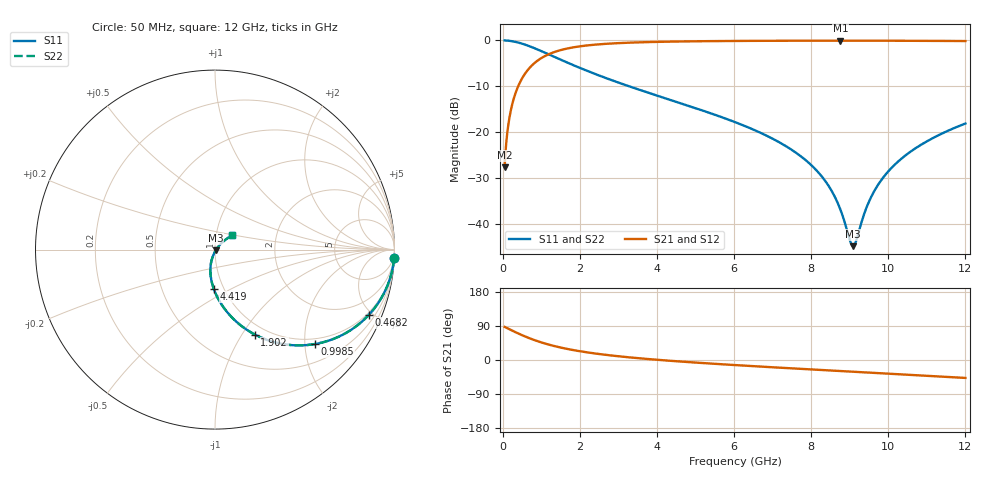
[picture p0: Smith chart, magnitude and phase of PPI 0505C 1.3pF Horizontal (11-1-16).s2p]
# MHz S MA R 50
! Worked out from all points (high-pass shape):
!   1601 points, 50 MHz to 12 GHz, reference 50 ohm
!   highest |S21| = -0.05 dB at 8.759 GHz (marker M1); lowest = -27.6 dB at 50 MHz (marker M2)
!   |S21| within 3 dB of the highest: 1.182 GHz to end of sweep
!   lowest |S11| = -44.8 dB at 9.087 GHz (marker M3), VSWR 1.01, Z = 50.5 - j0.307 ohm
!   |S11| at or under -10 dB: 3.281 GHz to end of sweep
!   |S22| runs from -44.8 to 0.0 dB; largest |S21 - S12| = 0
!   S11 on the Smith chart (normalised r, x): 50 MHz: 1, -45; 468.2 MHz: 0.87, -4.78; 998.5 MHz: 0.87, -2.23; 1.902 GHz: 0.88, -1.14; 4.419 GHz: 0.90, -0.41; 12 GHz: 1.20, +0.19
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50  0.9991 -2.6  0.0415 87.4  0.0415 87.4  0.9991 -2.6
147.0938  0.9926 -7.5  0.1213 82.5  0.1213 82.5  0.9926 -7.5
214.3125  0.9844 -10.8  0.1753 79.1  0.1753 79.1  0.9844 -10.8
468.25  0.9315 -22.9  0.363 67.0  0.363 67.0  0.9315 -22.9
998.5312  0.7665 -43.3  0.6407 46.6  0.6407 46.6  0.7665 -43.3
1902.25  0.5227 -64.9  0.85 24.9  0.85 24.9  0.5227 -64.9
2044.156  0.4938 -67.3  0.867 22.5  0.867 22.5  0.4938 -67.3
2888.125  0.3613 -78.4  0.9293 11.1  0.9293 11.1  0.3613 -78.4
4038.312  0.2479 -88.9  0.965 0.3  0.965 0.3  0.2479 -88.9
4419.219  0.2199 -91.7  0.9715 -2.6  0.9715 -2.6  0.2199 -91.7
6025  0.1289 -101.5  0.9869 -13.4  0.9869 -13.4  0.1289 -101.5
7205.062  0.07639 -106.7  0.9918 -20.4  0.9918 -20.4  0.07639 -106.7
8019.156  0.04318 -108.0  0.9933 -25.0  0.9933 -25.0  0.04318 -108.0
8444.875  0.02635 -105.5  0.9937 -27.4  0.9937 -27.4  0.02635 -105.5
8758.562  0.01438 -96.3  0.9938 -29.1  0.9938 -29.1  0.01438 -96.3
9005.031  0.006635 -61.2  0.9937 -30.5  0.9937 -30.5  0.006635 -61.2
9087.188  0.005742 -32.0  0.9937 -30.9  0.9937 -30.9  0.005742 -32.0
9161.875  0.006462 -4.7  0.9936 -31.4  0.9936 -31.4  0.006462 -4.7
9550.25  0.01949 38.7  0.9933 -33.5  0.9933 -33.5  0.01949 38.7
10013.31  0.038 44.5  0.9925 -36.1  0.9925 -36.1  0.038 44.5
10834.88  0.0724 44.1  0.9901 -40.7  0.9901 -40.7  0.0724 44.1
12000  0.1245 39.3  0.9842 -47.3  0.9842 -47.3  0.1245 39.3
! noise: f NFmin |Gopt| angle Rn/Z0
50  0.001017  0.9623  1.65  0.006095
1372  0.005841  0.7683  6.552  0.005116
2701  0.00922  0.7178  10.77  0.006406
4031  0.01221  0.6883  15.06  0.007486
5360  0.01502  0.669  19.34  0.008482
6682  0.01775  0.6562  23.53  0.009452
8012  0.02048  0.6483  27.67  0.01045
9341  0.02327  0.6443  31.71  0.0115
1.067e+04  0.02616  0.6436  35.65  0.01265
1.2e+04  0.0292  0.6458  39.48  0.01392
